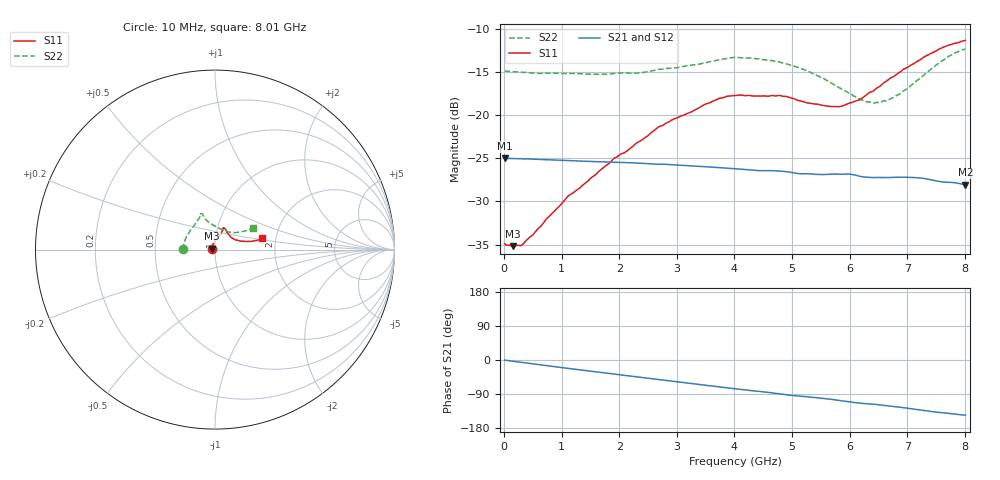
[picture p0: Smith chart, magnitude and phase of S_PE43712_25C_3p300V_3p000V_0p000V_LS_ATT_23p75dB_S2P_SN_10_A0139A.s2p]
! DEVICE ID: PE43712
! File Path: z:\PE43713\PE43713_CHAR_NOM_04292014\AMB\3p300\LS_ATT_23p75dB\PE43713_AMB_3p300V_3p000V_0p000V_LS_ATT_23p75dB_S2P_SN_10_A0139A.s2p
! Serial: 10
! Lot: A0139A
! Temp: 25C
! VDD: 3.300
! VSS: 0.000
! Control_Hi: 3.000
! Control_Lo: 0.000
! Attenuation Step: 23.75dB
! Port 1: RF1
! Port 2: RF2
! ThroughPath:1-2
! IDD: 0.0001473419
! ISS: -1.744e-007
#  Hz  S  RI  R  50
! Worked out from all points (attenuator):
!   801 points, 10 MHz to 8.01 GHz, reference 50 ohm
!   highest |S21| = -24.99 dB at 20 MHz (marker M1); lowest = -28.1 dB at 8.01 GHz (marker M2)
!   lowest |S11| = -35.2 dB at 160 MHz (marker M3), VSWR 1.04, Z = 48.4 + j0.524 ohm
!   |S11| at or under -10 dB: start of sweep to end of sweep
!   |S22| runs from -18.6 to -12.4 dB; largest |S21 - S12| = 0.0002
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1e7  -0.018 0.000676  0.0563 -0.000278  0.0563 -0.000253  -0.1806 0.0012
2e7  -0.0178 0.00122  0.0563 -0.000459  0.0563 -0.000469  -0.1804 0.00209
1.6e8  -0.0166 0.00541  0.056 -0.00336  0.056 -0.00335  -0.1784 0.0114
3.3e8  -0.015 0.00971  0.0555 -0.00676  0.0554 -0.00671  -0.176 0.0208
1.1e9  -0.0101 0.0322  0.0506 -0.0204  0.0506 -0.0204  -0.1622 0.0642
1.35e9  -0.00646 0.0384  0.0485 -0.0243  0.0484 -0.0243  -0.1562 0.0761
1.91e9  0.00505 0.056  0.0426 -0.0322  0.0426 -0.0322  -0.1378 0.1076
2.35e9  0.0169 0.0684  0.037 -0.0376  0.037 -0.0376  -0.1202 0.1284
2.68e9  0.0271 0.0809  0.0325 -0.0406  0.0325 -0.0406  -0.1066 0.1504
3.71e9  0.0447 0.1157  0.0166 -0.0469  0.0166 -0.0469  -0.0815 0.1918
4.01e9  0.0472 0.1214  0.0119 -0.0475  0.012 -0.0475  -0.0807 0.2005
4.76e9  0.0542 0.1183  0.000862 -0.0475  0.000904 -0.0475  -0.0668 0.1932
5.35e9  0.0686 0.0944  -0.00684 -0.0452  -0.00685 -0.0451  -0.0517 0.1676
5.64e9  0.08 0.0792  -0.0102 -0.0443  -0.0102 -0.0444  -0.0339 0.1527
5.87e9  0.0908 0.0672  -0.0136 -0.0434  -0.0135 -0.0434  -0.0156 0.1406
6.17e9  0.1094 0.0561  -0.0179 -0.0406  -0.0178 -0.0406  0.0132 0.1233
6.39e9  0.1269 0.0517  -0.0193 -0.0389  -0.0193 -0.0389  0.0379 0.1114
6.68e9  0.1549 0.0465  -0.0224 -0.0374  -0.0223 -0.0373  0.073 0.0991
7e9  0.1833 0.0458  -0.0264 -0.0348  -0.0263 -0.0347  0.1067 0.0945
7.55e9  0.2356 0.0519  -0.0309 -0.0275  -0.0309 -0.0274  0.171 0.1051
7.81e9  0.2537 0.0581  -0.0322 -0.0248  -0.0322 -0.0249  0.1975 0.1141
8.01e9  0.2638 0.0634  -0.0325 -0.0224  -0.0324 -0.0226  0.2104 0.1178
